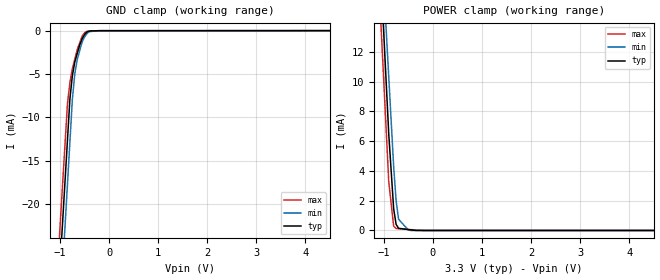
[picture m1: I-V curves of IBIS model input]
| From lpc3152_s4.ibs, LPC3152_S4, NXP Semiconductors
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[Model] input
Model_type Input
Vinl = 990.000mV
Vinh = 2.31000V
C_comp 887.000fF 880.000fF 894.000fF
| variable typ   min   max
[Voltage Range] 3.30000V 3.00000V 3.60000V
[POWER Clamp Reference] 3.30000V 3.00000V 3.60000V
[GND Clamp Reference] 0.00000V 0.00000V 0.00000V
[Temperature Range]   25   85   -40
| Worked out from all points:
|   GND clamp passes 1 mA (typ) near -0.56 V on its own axis
|   POWER clamp passes 1 mA (typ) near -0.78 V on its own axis
[GND Clamp]
-3.3V     -247mA     -258mA     -238.4mA
-850mV    -12.66mA   -17.74mA   -8.44mA
-800mV    -7.875mA   -12.84mA   -5.98mA
-750mV    -5.191mA   -7.936mA   -4.374mA
-700mV    -3.6mA     -4.96mA    -3.268mA
-650mV    -2.619mA   -3.316mA   -2.161mA
-600mV    -1.638mA   -2.304mA   -1.397mA
-550mV    -925.7uA   -1.292mA   -633.6uA
-450mV    -147.8uA   -317.7uA   -56.84uA
-400mV    -35.53uA   -109.1uA   -44.84uA
-200mV    -2.215uA   -2.738uA   -2.802uA
6.6V      6.05uA     12.1uA     7.423uA
[POWER Clamp]
-3.3V     166.2mA    154.9mA    162.9mA
-1.1V     19.79mA    22.37mA    16.57mA
-1.05V    16.46mA    19.36mA    13.25mA
-900mV    6.474mA    10.33mA    3.274mA
-800mV    1.457mA    4.302mA    287.1uA
-750mV    410uA      2.004mA    135.4uA
-700mV    144.5uA    754.6uA    122.5uA
-500mV    61.94uA    28.52uA    70.93uA
-450mV    41.29uA    27.2pA     58.04uA
-150mV    0A         0A         0A
6.6V      0A         0A         0A
